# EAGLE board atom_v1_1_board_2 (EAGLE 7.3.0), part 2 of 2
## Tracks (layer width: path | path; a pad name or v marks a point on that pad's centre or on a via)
+3V3  (via drill 0.3)
  Top 0.152: 21.79,90.22 20.27,90.22 19.96,89.92 C9.+ 19.89,89.84 19.89,87.4 16.08,83.59 v16.08,83.21 | 21.79,90.22 25,90.22 C7.1 | 21.79,90.22 21.79,95.1 23.09,96.39 IC4.2 25.45,96.55 v26.29,97.38 | 12.35,75.89 13.34,75.89 15.32,77.88 17.76,77.88 18.52,78.64 SW3.B 18.59,78.72 v20.8,78.72 25.3,78.72 SW3.B' | 12.35,75.89 5.49,75.89 4.72,76.66 4.42,76.66 R45.2 | 68.89,78.03 68.89,79.25 R53.2 | 68.89,78.03 68.89,77.27 R52.2 68.81,77.19 68.5,77.19 v66.91,75.59 | 68.89,78.03 71.17,78.03 71.32,77.88 71.32,76.58 70.64,75.89 70.64,75.21 C39.1 70.56,75.13 v70.56,74.07 | 65.42,74.11 66.52,73 67.36,73 IC12.27 | 65.42,74.11 65.15,74.37 59.21,74.37 58.37,75.21 57.99,75.21 C38.1 | v58.29,73.08 58.83,73.61 59.82,73.61 IC12.1 | v57.46,74.07 57.46,74.75 57.84,75.13 C38.1 | v65.46,74.14 65.42,74.11 | 43.51,76.2 43.51,74.98 43.59,74.91 IC10.64 | 43.51,76.2 43.51,77.19 C21.1 43.51,77.27 v43.51,78.41 | C34.1 43.44,65.08 41.68,65.08 41.53,65.23 IC10.48 41.45,65.3 41.45,65.84 v40.84,66.45 | 12.35,75.89 12.35,73.99 12.5,73.84 21.95,73.84 23.7,75.59 27.05,75.59 29.11,73.53 29.11,73.46 C22.1 29.11,73.38 30.71,73.38 31.17,73.84 31.78,73.84 IC10.19 31.85,73.84 32.46,73.84 v33,73.3 | v33.07,63.17 32.92,63.02 32.01,63.02 C33.1 | v33,67.36 31.85,67.36 IC10.32 | 57.91,76.2 57.91,75.21 C38.1 | 57.91,76.2 57.91,77.19 C36.1 | v57,76.2 57.91,76.2 | 43.51,76.2 v44.35,76.2
  Bottom 0.152: v16.08,83.21 16.08,80.16 17.53,78.72 v20.8,78.72 | v58.29,73.08 58.29,73.23 v57.46,74.07 | v65.46,74.14 v66.91,75.59 | v33.07,63.17 33.07,67.28 v33,67.36 32.31,68.05 32.31,70.56 32.77,71.02 33,71.02 | v40.84,66.45 39.32,66.45 34.75,71.02 33,71.02 | v33,73.3 33,71.02 | v57,76.2 50.45,76.2 50.06,75.82 44.73,75.82 v44.35,76.2 | v43.51,78.41 43.51,81.38 45.03,82.91 45.03,83.06 JP1.1 | v26.29,97.38 30.33,97.38 34.14,101.19 52.81,101.19 53.34,101.73 66.91,101.73 70.56,98.07 v70.56,74.07
+3V3_A  (via drill 0.3)
  Top 0.152: C23.1 10.9,69.04 10.9,65.61 10.36,65.08 8.15,65.08 7.85,64.77 7.85,62.71 10.9,59.66 10.9,57.45 C29.1 10.9,57.38 v10.9,56.16 | v7.16,52.43 8.23,51.36 8.69,51.36 IC6.4 | v11.81,64.85 13.87,66.9 14.4,66.9 IC9.8 14.48,66.98 20.96,73.46 v23.47,73.46 | 32.01,78.94 32.01,79.25 C18.1 32.01,78.94 | 32.01,78.94 32.01,77.27 C17.1 | 32.01,78.94 34.82,78.94 | 34.82,78.94 35.13,78.94 35.59,78.49 35.59,78.03 35.51,77.95 35.51,77.11 IC10.13 | IC2.2 52.81,96.47 50.29,93.95 50.29,93.34 50.9,92.73 50.9,90.3 C8.1 50.83,90.3 v49.91,89.38 49.91,88.54 49.23,87.86 49.23,86.03 53.72,81.53 v53.72,73.08 | v34.82,79.25 34.82,78.94 | v54.26,89.84 C10.+ | 60.69,57.11 58.98,55.4 58.98,49.91 59.44,49.45 61.65,49.45 61.8,49.61 61.8,50.52 61.04,51.28 60.58,51.28 IC13.4 | 60.69,57.11 61.42,57.84 61.88,57.84 62.26,57.45 62.71,57.45 C51.1 | C48.1 57.91,61.49 57.91,63.48 C46.1 57.99,63.48 58.14,63.48 59.4,64.73 | 59.4,64.73 59.82,65.15 IC12.14 | v58.29,68.35 58.98,69.04 59.82,69.04 IC12.8 | 59.4,64.73 v58.29,65.84 | v60.66,57.23 60.66,57.15 60.69,57.11 | v48.31,39.55 47.17,39.55 IC3.16 | v48.31,40.92 45.87,40.92 45.84,40.96 | 45.84,40.96 45.19,41.6 C13.1 | IC5.16 47.17,30.33 49.15,30.33 49.61,30.79 49.61,31.24 48.39,32.46 45.19,32.46 C37.1 | 45.84,40.96 45.8,40.92 45.8,36.04 45.19,35.43 45.19,32.54 C37.1 | v53.27,36.27 57,32.54 57.23,32.54 JP102.1 | v36.88,56.01 36.88,57.38 C32.1 | v36.88,54.1 36.88,53.11 35.13,51.36 34.67,51.36 IC7.4 35.43,51.59 v36.27,50.75 | 32.5,41.11 32.01,41.6 C6.1 | 32.5,41.11 33.91,39.7 33.91,39.55 IC8.16 33.99,39.47 34.37,39.47 35.81,38.02 35.81,32.46 | C16.1 32.01,32.46 33.91,30.56 33.91,30.4 IC11.16 33.99,30.33 34.44,30.33 34.48,30.29
  Top 0.152: 34.48,30.29 36.42,28.35 36.42,26.29 28.73,18.59 17.76,18.59 14.78,15.62 13.87,15.62 R60.2 | 35.81,32.46 35.81,31.62 34.48,30.29 | 32.5,41.11 v33.07,41.68 | 35.81,32.46 40.92,32.46 42.75,30.63 43.74,30.63 45.19,32.08 45.19,32.38 C37.1
  Bottom 0.152: v7.16,52.43 v10.9,56.16 11.81,57.07 v11.81,64.85 | v54.26,89.84 50.37,89.84 v49.91,89.38 45.26,89.38 35.13,79.25 v34.82,79.25 34.44,78.87 28.88,78.87 v23.47,73.46 | v48.31,39.55 v48.31,40.92 52.81,40.92 53.23,40.5 | v53.27,36.27 53.27,40.46 53.23,40.5 | 53.23,40.5 53.27,40.54 53.8,40.54 60.66,47.4 v60.66,57.23 60.66,57.68 58.29,60.05 v58.29,65.84 v58.29,68.35 58.29,68.5 v53.72,73.08 | v36.88,54.1 v36.88,56.01 | v36.27,50.75 36.27,46.25 33.07,43.05 v33.07,41.68
ADC_ADDR_0  (via drill 0.3)
  Top 0.152: v32.84,27.13 33.91,27.13 IC11.11 | v32.84,35.59 33.53,36.27 33.91,36.27 IC8.11 | v45.34,27.13 47.09,27.13 IC5.11 | v48.24,35.97 47.93,36.27 47.17,36.27 IC3.11 | v36.5,75.59 36.88,75.21 38.71,75.21 39.93,76.43 39.93,77.04 IC10.4 | v29.41,64.01 29.41,62.41 33.53,58.29 34.9,58.29 36.12,57.07 36.12,55.85 38.1,53.87 v38.1,50.75
  Bottom 0.152: v32.84,35.59 32.84,32.31 | 32.84,32.31 v32.84,27.13 | 32.84,32.31 34.67,32.31 38.63,28.35 40.08,28.35 40.69,28.96 40.69,29.41 43.28,32 43.74,32 44.2,31.55 44.2,31.09 42.98,29.87 42.98,26.9 43.44,26.44 43.89,26.44 44.58,27.13 v45.34,27.13 46.71,28.5 46.71,34.44 v48.24,35.97 48.16,35.97 47.02,37.11 47.02,41.83 v38.1,50.75 | v36.5,75.59 34.06,75.59 33.53,75.06 33.38,75.06 31.01,72.69 31.01,65.61 v29.41,64.01
ADC_ADDR_1  (via drill 0.3)
  Top 0.152: v35.05,26.82 34.75,26.52 33.99,26.52 IC11.10 | v34.44,31.62 34.44,34.44 34.67,34.67 34.67,35.28 34.37,35.59 33.99,35.59 IC8.10 | v46.03,26.44 47.09,26.44 IC5.10 | v48.24,34.98 47.63,35.59 47.17,35.59 IC3.10 | v40.54,70.94 40.54,77.04 IC10.3 | v50.06,64.47 50.75,63.78 50.75,56.77 v47.93,53.95 | v40.39,26.82 v38.48,26.82
  Bottom 0.152: v34.44,31.62 34.44,27.58 35.05,26.98 v35.05,26.82 v38.48,26.82 | v40.54,70.94 40.54,70.18 45.03,65.68 48.84,65.68 v50.06,64.47 | v47.93,53.95 47.93,44.73 47.32,44.12 47.32,37.8 48.92,36.2 48.92,35.66 v48.24,34.98 47.55,34.29 47.55,28.88 46.03,27.36 v46.03,26.44 45.72,26.14 43.28,26.14 42.6,26.82 v40.39,26.82
ADC_ADDR_2  (via drill 0.3)
  Top 0.152: v32.84,26.14 33.07,25.91 33.91,25.91 IC11.9 | v32.16,33.68 32.62,33.68 33.91,34.98 IC8.9 | v48.24,26.21 47.93,25.91 47.17,25.91 IC5.9 | v48.24,33.91 47.17,34.98 IC3.9 | v44.35,84.89 41,81.53 41,77.11 IC10.2 | v54.41,71.48 v54.41,81.61 | v52.58,40.23 v53.57,41.22 | v40.08,24 45.19,24 v45.42,23.77
  Bottom 0.152: v32.16,33.68 32.16,26.82 v32.84,26.14 37.95,26.14 v40.08,24 | 48.24,33.83 v48.24,26.21 45.8,23.77 v45.42,23.77 | v44.35,84.89 51.13,84.89 v54.41,81.61 | v54.41,71.48 54.41,69.95 57.61,66.75 57.61,52.96 59.67,50.9 59.67,47.17 53.72,41.22 v53.57,41.22 | v52.58,40.23 52.58,38.18 48.24,33.83 | 48.24,33.83 v48.24,33.91
ADC_BANK_0  (via drill 0.3)
  Top 0.152: v27.2,27.05 27.28,27.13 28.27,27.13 IC11.6 | v42.52,51.44 43.97,51.44 44.43,51.89 44.43,52.96 44.73,53.26 49.38,53.26 52.27,56.16 52.58,56.16 54.79,58.37 54.79,65.91 v58.29,69.42 | v48.16,73.99 45.57,71.4 43.66,71.4 IC10.57
  Bottom 0.152: v27.2,27.05 27.2,28.88 25.83,30.25 25.83,38.48 27.28,39.93 31.39,39.93 32.39,40.92 32.39,47.78 36.04,51.44 v42.52,51.44 | v58.29,69.42 53.72,73.99 v48.16,73.99
ADC_BANK_1  (via drill 0.3)
  Top 0.152: v26.52,38.25 26.52,37.34 27.51,36.35 28.27,36.35 IC8.6 | v38.02,45.11 45.95,45.11 47.93,47.09 47.93,50.9 v49.3,52.27 | v55.48,58.45 v51.05,54.03 | v46.56,73.3 45.19,71.93 43.66,71.93 IC10.58
  Bottom 0.152: v26.52,38.25 31.17,38.25 v38.02,45.11 | v51.05,54.03 v49.3,52.27 | v55.48,58.45 55.48,68.43 50.6,73.3 v46.56,73.3
ADC_BANK_2  (via drill 0.3)
  Top 0.152: v39.7,29.34 39.7,28.57 41.07,27.2 41.45,27.2 IC5.6 | v43.28,42.82 47.4,42.82 v51.36,46.79 | v52.35,65 v52.35,56.84 | v44.96,72.62 44.5,72.62 44.27,72.39 43.66,72.39 IC10.59
  Bottom 0.152: v39.7,29.34 39.7,34.37 42.6,37.26 42.6,42.14 v43.28,42.82 | v51.36,46.79 51.36,47.24 52.35,48.23 v52.35,56.84 | v52.35,65 52.35,65.15 52.96,65.76 52.96,69.88 50.22,72.62 v44.96,72.62
ADC_BANK_3  (via drill 0.3)
  Top 0.152: v40.31,36.35 41.45,36.35 IC3.6 | v36.65,42.75 35.74,42.75 33.68,44.81 30.25,44.81 29.41,45.64 29.41,47.24 28.8,47.85 v28.8,48.84 | v41.07,57.23 45.57,57.23 49.07,60.73 49.07,66.98 v49.45,67.36 | v42.44,72.77 42.98,73.3 43.59,73.3 IC10.61
  Bottom 0.152: v40.31,36.35 40.31,39.09 v36.65,42.75 | v28.8,48.84 37.19,57.23 v41.07,57.23 | v49.45,67.36 47.85,67.36 v42.44,72.77
ADC_BLOW_SHAPE  (via drill 0.3)
  Top 0.152: R12.1 19.28,46.25 19.28,48.23 C15.2 | v33.07,77.34 33.3,77.11 33.91,77.11 IC10.16 | v24.46,73.53 24.46,72.62 25.83,71.25 25.83,70.79 22.86,67.82 v22.86,66.22 | v20.5,49.53 19.28,48.31 C15.2 | IC6.8 14.94,47.55 15.47,47.55 16.99,49.07 18.44,49.07 19.2,48.31 C15.2
  Bottom 0.152: v33.07,77.34 28.27,77.34 v24.46,73.53 | v22.86,66.22 22.86,51.89 v20.5,49.53
ADC_BLOW_TIMBRE  (via drill 0.3)
  Top 0.152: 6.1,47.47 6.1,48.23 C27.2 | 6.1,47.47 6.1,47.24 | 6.1,47.24 6.1,46.25 R35.1 | v39.85,74.91 31.85,74.91 IC10.17 | v16.77,80.39 12.96,80.39 v11.96,79.4 | 6.1,47.24 v5.18,47.24 | 6.1,47.47 8.69,47.47 IC6.7
  Bottom 0.152: v39.85,74.91 42.75,74.91 43.36,75.51 57.23,75.51 59.67,77.95 59.67,87.02 56.16,90.53 40.92,90.53 30.79,80.39 v16.77,80.39 | v11.96,79.4 11.96,65.91 5.18,59.13 v5.18,47.24
ADC_BOW_TIMBRE  (via drill 0.3)
  Top 0.152: R11.1 19.28,55.17 | 19.28,55.17 19.28,54.41 C14.2 | v33,76.35 33.15,76.2 34.22,76.2 34.44,76.43 34.44,77.04 IC10.15 | v25.15,71.02 25.15,70.79 v21.26,66.9 | v19.51,57.53 19.51,56.62 R11.1 | R11.1 | 19.28,55.17 14.94,55.17 IC6.14
  Bottom 0.152: v33,76.35 31.85,76.35 28.73,73.23 27.36,73.23 v25.15,71.02 | v21.26,66.9 20.35,66.9 19.51,66.06 v19.51,57.53
ADC_BRIGHTNESS  (via drill 0.3)
  Top 0.152: C42.2 71.1,48.23 71.1,46.25 R49.1 71.02,46.18 71.02,45.64 69.8,44.42 69.34,44.42 67.51,46.25 67.51,46.71 66.75,47.47 IC13.8 66.68,47.55 66.37,47.85 v65.08,47.85 | v33,70.33 31.85,70.33 IC10.26 | v58.98,47.4 59.67,46.71 v64.39,46.71
  Bottom 0.152: v33,70.33 33.15,70.33 39.02,64.47 44.73,64.47 51.66,57.53 52.58,57.53 58.98,51.13 v58.98,47.4 | v64.39,46.71 64.39,47.17 v65.08,47.85
ADC_DAMPING  (via drill 0.3)
  Top 0.152: R18.1 43.51,46.25 43.51,48.23 C20.2 43.44,48.23 v42.52,49.15 42.67,48.92 41.3,47.55 40.84,47.55 IC7.8 | v37.95,72.31 31.85,72.31 IC10.22 | v50.06,63.48 50.06,57.07 v46.94,53.95
  Bottom 0.152: v37.95,72.31 44.88,65.38 48.16,65.38 v50.06,63.48 | v46.94,53.95 46.94,53.57 v42.52,49.15
ADC_FM  (via drill 0.3)
  Top 0.152: 19.43,68.43 17.45,68.43 C25.2 17.38,68.35 17.38,68.12 14.94,65.68 14.48,65.68 IC9.7 | v30.25,75.67 35.66,75.67 36.42,76.43 36.42,77.04 IC10.11 | v24,72.16 23.17,72.16 19.43,68.43 | 19.43,68.43 R28.1
  Bottom 0.152: v30.25,75.67 27.51,75.67 v24,72.16
ADC_GEOMETRY  (via drill 0.3)
  Top 0.152: 32.01,47.47 32.01,48.23 C28.2 31.93,48.31 v32.84,49.23 | 32.01,47.47 32.01,46.25 R29.1 | v35.36,69.49 33,71.86 31.85,71.86 IC10.23 | v46.1,64.01 46.1,62.48 44.2,60.58 v42.29,60.58 | 32.01,47.47 34.6,47.47 IC7.7
  Bottom 0.152: v35.36,69.49 35.36,68.58 39.17,64.77 45.34,64.77 v46.1,64.01 | v42.29,60.58 42.29,55.17 38.86,51.74 35.36,51.74 v32.84,49.23
ADC_POSITION  (via drill 0.3)
  Top 0.152: C41.2 71.1,54.41 71.1,56.39 R48.1 71.02,56.39 71.02,57.23 66.68,61.57 64.16,61.57 63.32,60.73 63.32,60.43 63.25,60.35 v59.67,60.35 | v39.85,72.62 36.04,68.81 35.13,68.81 34.67,69.27 34.67,69.57 33.22,71.02 32.77,71.02 32.69,70.94 31.85,70.94 IC10.25 | v61.65,57.15 63.63,55.17 66.68,55.17 IC13.14
  Bottom 0.152: v39.85,72.62 41.38,72.62 43.44,74.68 53.95,74.68 59.67,68.96 v59.67,60.35 59.67,59.13 v61.65,57.15
ADC_POTS  (via drill 0.3)
  Top 0.152: v38.18,80.92 37.72,81.38 TP1.P$1 37.72,87.55 41.84,91.67 43.59,91.67 43.89,91.97 43.89,93.12 44.05,93.27 45.26,93.27 48.92,89.61 48.92,85.88 50.98,83.82 v50.98,70.41 | v36.81,80.01 37.26,80.01 37.95,79.32 37.95,77.11 IC10.8 | v27.13,29.87 27.89,29.11 28.27,29.11 IC11.3 | v27.2,37.57 27.81,38.18 28.27,38.18 IC8.3 | v38.25,31.77 41.15,31.77 42.29,30.63 42.29,29.49 41.91,29.11 41.53,29.11 IC5.3 | v43.28,37.19 42.33,38.14 | 42.33,38.14 42.29,38.18 41.53,38.18 IC3.3 | v51.66,67.67 49.38,65.38 49.38,57.3 v48.62,56.54 | v48.62,47.32 44.81,43.51 43.05,43.51 42.37,42.82 42.37,38.18 42.33,38.14
  Bottom 0.152: v38.18,80.92 37.72,80.92 v36.81,80.01 | v27.13,29.87 27.13,34.75 26.44,35.43 26.44,36.8 v27.2,37.57 27.2,37.49 27.43,37.26 32.77,37.26 v38.25,31.77 38.25,29.87 39.47,28.65 39.93,28.65 40.39,29.11 40.39,29.57 43.28,32.46 v43.28,37.19 | v50.98,70.41 50.98,68.66 51.66,67.97 v51.66,67.67 | v48.62,47.32 v48.62,56.54
ADC_PRESSURE  (via drill 0.3)
  Top 0.152: C26.2 4.34,54.41 4.34,56.39 R34.1 4.65,56.39 5.49,57.23 6.63,57.23 IC6.1 9.14,54.71 v10.36,54.71 | v34.9,78.26 34.9,77.11 IC10.14 | v28.8,72.24 28.2,72.24 v23.55,67.59
  Bottom 0.152: v34.9,78.26 34.9,77.34 33.22,75.67 32.23,75.67 v28.8,72.24 | v23.55,67.59 20.57,67.59 12.12,59.13 12.12,56.46 v10.36,54.71
ADC_SPACE  (via drill 0.3)
  Top 0.152: R73.1 56.16,46.25 56.16,48.23 C50.2 | v33.07,69.19 32.46,69.8 31.85,69.8 IC10.27 | v51.36,48.62 55.7,48.62 56.08,48.23 C50.2 | IC13.7 60.5,47.55 59.97,47.55 58.45,49.07 57,49.07 56.24,48.31 C50.2
  Bottom 0.152: v33.07,69.19 33.07,68.2 36.42,64.85 36.42,63.78 36.88,63.32 37.64,63.32 38.18,63.86 39.93,63.86 46.56,57.23 48.84,57.23 51.74,54.33 51.74,49 v51.36,48.62
ADC_STRIKE_SHAPE  (via drill 0.3)
  Top 0.152: 30.25,56.39 30.25,55.17 | 30.25,55.17 30.25,54.41 C30.2 | v27.13,66.22 28.2,67.28 28.2,70.33 31.17,73.3 31.78,73.3 IC10.20 | 30.25,56.39 v27.13,59.51 | 30.25,56.39 R46.1 | 30.25,55.17 34.6,55.17 IC7.1
  Bottom 0.152: v27.13,59.51 v27.13,66.22
ADC_STRIKE_TIMBRE
  Top 0.152: C19.2 43.51,54.41 43.51,56.39 R17.1 40.77,56.39 | 40.77,56.39 40.77,55.17 IC7.14 | 40.77,56.39 40.77,56.62 33.53,63.86 31.7,63.86 31.17,64.39 31.17,66.22 29.57,67.82 29.57,71.25 31.17,72.85 31.78,72.85 IC10.21
ADC_V_OCT  (via drill 0.3)
  Top 0.152: 4.19,68.43 6.17,68.43 C24.2 6.25,68.35 7.62,66.98 9.14,66.98 IC9.1 | v32.46,82.98 36.96,78.49 36.96,77.11 IC10.10 | v10.21,84.51 3.28,77.57 3.28,69.34 4.19,68.43 | 4.19,68.43 R27.1
  Bottom 0.152: v32.46,82.98 17.22,82.98 15.7,84.51 v10.21,84.51
AREF_-10
  Top 0.152: R32.2 4.34,50.29 4.34,52.27 R31.2 4.34,52.35 3.58,53.11 3.58,57 6.13,59.55 | 6.13,59.55 6.17,59.59 6.17,62.64 R37.2 | 30.25,50.29 30.25,52.27 R41.2 | 19.28,51.51 19.28,52.27 R14.2 19.28,52.35 20.19,53.26 20.19,57.76 17.45,60.5 17.45,62.64 R38.2 | 19.28,51.51 R15.2 | R15.2 29.49,50.29 | 29.49,50.29 30.25,50.29 | 30.25,50.29 R42.2 | R15.2 | 19.28,51.51 16.99,51.51 16.61,51.89 13.87,51.89 13.64,52.12 13.64,52.35 6.48,59.51 6.17,59.51 6.13,59.55 | C2.1 70.64,92.96 70.64,88.32 IC1.2 70.64,88.24 70.64,85.88 R2.2 70.56,85.8 R1.2 70.64,83.82 70.64,80.62 74.3,76.96 74.3,56.16 71.25,53.11 71.02,53.11 70.98,53.07 | R56.2 71.1,50.29 71.1,52.27 R55.2 71.02,52.35 71.02,53.03 70.98,53.07 | 45.19,50.29 45.19,52.27 R20.2 45.26,52.27 45.95,52.96 49.53,52.96 52.2,50.29 R70.2 56.24,50.29 56.24,53.72 60.73,58.22 63.4,58.22 63.55,58.06 63.55,56.92 63.86,56.62 65.08,56.62 65.69,57.23 69.95,57.23 70.18,57 70.18,53.87 70.98,53.07 | 29.49,50.29 29.49,47.62 30.1,47.02 30.86,47.02 31.17,46.71 31.17,45.64 31.39,45.41 35.43,45.41 35.81,45.8 42.52,45.8 42.9,45.41 45.8,45.41 45.95,45.57 45.95,49.53 45.19,50.29 | 45.19,50.29 R21.2
BOOT_FLASH  (via drill 0.3)
  Top 0.152: R50.2 17.3,76.66 17.3,75.97 18.52,74.75 SW3.A 18.59,74.68 20.65,74.68 v20.8,74.52 | v48.16,77.8 48.16,76.73 44.35,72.92 43.66,72.92 IC10.60 | v27.59,72.54 25.38,74.75 SW3.A'
  Bottom 0.152: v48.16,77.8 48.16,78.26 51.28,81.38 51.28,83.13 50.52,83.9 43.05,83.9 35.05,75.89 33.91,75.89 33.38,75.36 32.84,75.36 29.03,71.55 28.58,71.55 v27.59,72.54 27.59,72.47 25.45,70.33 24.92,70.33 23.32,71.93 23.32,72.01 v20.8,74.52
GATE  (via drill 0.3)
  Top 0.152: Q2.3 13.87,11.28 13.87,13.87 R60.1 13.95,13.87 v16,15.93 | v30.25,70.41 31.17,71.32 31.78,71.32 IC10.24 | v26.06,66.22 v27.51,67.67 | v20.5,44.81 20.5,44.65 16,40.16 v16,34.52
  Bottom 0.152: v27.51,67.67 v30.25,70.41 | v26.06,66.22 26.06,50.37 v20.5,44.81 | v16,15.93 v16,34.52
GND  (via drill 0.3)
  Top 0.152: IC12.15 67.44,65.15 69.04,63.55 69.34,63.55 C47.2 69.42,63.48 69.72,63.48 70.49,62.71 72.09,62.71 72.92,63.55 72.92,65.23 68.31,69.84 | 67.78,74.11 67.36,73.69 IC12.28 67.29,73.69 66.83,73.69 61.49,79.02 56.16,79.02 | 67.78,74.11 68.81,75.13 C39.2 | 68.31,69.84 69.65,71.17 69.65,72.24 67.78,74.11 | 68.31,69.84 68.28,69.8 67.44,69.8 IC12.22 67.36,69.72 67.36,69.11 IC12.21 67.29,69.11 62.71,69.11 60.81,67.21 59.89,67.21 IC12.11 59.82,67.13 58.67,67.13 56.24,64.69 56.24,63.55 C46.2 56.16,63.48 56.16,61.49 C48.2 56.24,61.42 57.99,59.66 64.54,59.66 | 64.54,59.66 64.54,60.12 65.38,60.96 C52.- | 64.54,59.66 64.54,57.45 C51.2 | C35.2 45.19,63.02 45.19,65 C34.2 45.19,65.08 45.19,66.22 48.69,69.72 51.89,69.72 52.96,70.79 54.64,70.79 56.16,72.31 56.16,75.13 C38.2 56.16,75.21 56.16,77.19 C36.2 56.16,77.27 56.16,79.02 | IC10.63 44.27,74.37 45.11,75.21 45.11,77.19 C21.2 45.19,77.27 45.19,78.49 46.03,79.32 46.03,79.78 44.27,81.53 44.27,83.44 44.73,83.9 45.57,83.9 46.33,83.13 JP1.3 46.41,83.13 47.63,83.13 | 68.81,89.92 68.81,88.32 IC1.1 | 68.81,89.92 68.81,92.96 C2.2 | 63.63,89.92 68.81,89.92 | 52.47,88.51 56.01,84.96 C10.- 56.01,84.89 56.16,84.73 56.16,79.02 | 52.47,88.51 52.43,88.54 50.98,88.54 C8.2 50.98,88.47 50.14,87.63 v50.14,87.48 | 54.26,91.82 54.26,90.75 52.5,89 52.5,88.54 52.47,88.51 | 54.26,91.82 54.26,97.23 52.88,98.6 52.88,98.75 IC2.1 52.81,98.83 49.07,98.83 48.46,99.44 42.06,99.44 40.39,97.77 P1.4 | 63.63,89.92 58.52,89.92 56.62,91.82 54.26,91.82 | 63.63,89.92 C1.+ | C31.2 30.25,65 30.25,63.02 C33.2 30.33,62.94 30.63,62.94 34.98,58.6 37.26,58.6 38.48,57.38 C32.2 38.56,57.38 38.56,53.72 38.48,53.65 38.48,53.19 39.09,52.58 IC7.12 40.84,52.58 40.84,51.36 IC7.11 40.84,51.28 40.84,50.06 IC7.10 40.77,50.06 34.67,50.06 IC7.5 34.6,50.06 34.22,50.06 33.38,50.9 33.38,51.74 34.22,52.58 IC7.3
  Top 0.152: v30.33,68.5 31.17,69.34 31.78,69.34 IC10.28 | 30.33,65.53 30.33,65.08 C31.2 | 30.33,65.53 v30.33,66.14 | 13.37,53.68 14.48,52.58 IC6.12 | 13.37,53.68 12.73,54.33 12.73,57.38 C29.2 12.65,57.45 12.65,63.17 | 10.71,64.96 10.14,64.39 IC9.3 | 10.71,64.96 12.65,66.9 12.65,69.04 C23.2 12.65,69.11 7.47,74.3 7.47,74.68 SW2.A 7.39,74.75 4.88,74.75 3.58,76.05 3.58,77.42 9.98,83.82 10.44,83.82 11.96,85.34 C3.- | IC9.3 9.22,63.17 IC9.4 | IC9.3 | 12.65,63.17 12.5,63.17 10.71,64.96 | 12.65,63.17 14.4,63.17 IC9.5 14.48,63.17 14.94,63.17 15.77,64.01 15.77,64.16 17.15,65.53 30.33,65.53 | 30.33,65.53 C31.2 | SW2.A' 14.25,74.75 15.47,75.97 15.47,76.66 R50.1 15.55,76.73 15.85,76.73 16.61,77.5 27.74,77.5 29.15,76.09 | 29.15,76.09 30.25,77.19 C17.2 30.25,77.27 30.25,79.25 C18.2 30.33,79.25 31.13,80.05 | 29.15,76.09 29.11,76.05 29.11,75.06 C22.2 29.19,75.06 29.87,74.37 31.78,74.37 IC10.18 | 31.13,80.05 31.17,80.09 34.9,80.09 35.97,79.02 35.97,77.11 IC10.12 | C3.- 12.35,84.96 15.24,82.07 C4.2 15.32,81.99 16.23,81.08 17.68,81.08 19.89,83.29 19.89,84.89 C9.- 19.96,84.96 23.55,88.54 25,88.54 C7.2 | C3.- 12.35,85.04 11.43,85.95 11.43,89.53 5.41,95.56 JP2.1 | 40.31,95.25 42.9,92.66 42.9,92.51 C12.1 | 40.31,95.25 40.31,97.77 P1.4 | 40.31,95.25 P1.3 | 37.72,97.77 35.2,97.77 | P1.5 36.92,94.45 | 36.92,94.45 36.88,94.41 36.88,92.51 C5.2 | 35.2,95.25 35.97,94.49 36.88,94.49 36.92,94.45 | 35.2,95.25 35.2,97.77 | 35.2,97.77 P1.8 | 35.2,95.25 P1.7 35.13,95.25 32.54,92.66 32.54,92.51 C11.1 32.54,92.73 31.93,92.73 31.39,93.27 28.2,93.27 25.8,90.87 | 37.72,97.77 40.23,97.77 P1.4 | 37.72,97.77 P1.6 | IC4.1 23.09,93.57 25.8,90.87
  Top 0.152: 25.8,90.87 25.83,90.83 25.83,89.38 25.07,88.62 C7.2 | 31.13,80.05 31.09,80.09 31.09,82.37 25,88.47 C7.2 | 47.55,5.87 47.55,7.09 C54.2 | 47.55,5.87 47.55,5.11 R74.1 | 47.55,5.87 44.58,5.87 44.27,5.56 44.27,3.81 43.51,3.05 R59.1 42.52,3.05 40.39,5.18 IC14.5 40.31,5.18 38.63,3.5 38.63,3.05 C45.1 38.56,3.05 37.57,2.06 36.2,2.06 33.26,4.99 | 33.26,4.99 33.6,5.33 33.6,5.64 34.44,6.48 IC14.3 | 33.26,4.99 32.04,3.77 | 32.04,3.77 32.01,3.73 32.01,3.05 R69.1 | 27.89,5.87 27.89,7.09 C57.2 27.97,7.16 27.97,8.23 28,8.27 | 27.89,5.87 27.89,5.11 R87.1 | 28,8.27 30.86,11.12 36.81,11.12 C44.2 36.88,11.2 v36.88,14.48 | Q2.2 14.86,8.99 17.15,8.99 17.83,8.31 27.97,8.31 28,8.27 | 27.89,5.87 30.86,5.87 31.01,5.71 31.01,4.65 31.85,3.81 32.01,3.81 32.04,3.77 | IC6.10 14.94,50.06 14.94,51.28 IC6.11 14.86,51.28 v13.26,51.28 9.98,51.28 | 9.98,51.28 9.98,51.74 9.14,52.58 IC6.3 | 9.98,51.28 9.98,50.83 9.22,50.06 8.76,50.06 IC6.5 9.3,50.06 9.98,49.38 9.98,47.02 5.26,42.29 5.26,40.16 JP3.1 | IC5.7 41.53,26.44 41.53,25.91 IC5.8 41.45,25.83 v40.39,25.83 | IC11.8 28.27,25.91 28.27,26.44 IC11.7 28.35,26.52 28.73,26.52 30.02,27.81 31.47,27.81 | 31.47,27.81 33.91,27.81 IC11.12 33.99,27.81 v35.13,27.81 | 31.47,27.81 31.47,28.8 30.33,29.95 30.33,32.46 C16.2 | IC8.8 28.27,35.05 28.27,35.59 IC8.7 28.35,35.66 28.73,35.66 29.03,35.97 29.03,36.58 28.73,36.88 28.35,36.88 IC8.5 28.27,36.96 28.27,37.57 IC8.4 28.35,37.64 28.73,37.64 29.03,37.95 29.03,38.56 28.73,38.86 28.35,38.86 IC8.2 | IC8.2 28.27,38.94 28.27,39.47 IC8.1 28.35,39.55 30.25,41.45 30.25,41.6 C6.2 30.33,41.68 30.56,41.68 31.32,42.44 33.3,42.44 40.08,35.66 41.45,35.66 IC3.7
  Top 0.152: IC3.7 41.53,35.59 41.53,35.05 IC3.8 41.53,34.98 43.44,33.07 43.44,32.54 C37.2 43.51,32.46 v43.51,31.32 | IC3.7 41.61,35.59 42.6,35.59 43.97,36.96 43.97,37.41 43.51,37.87 43.51,41.6 C13.2 43.59,41.6 43.74,41.6 44.58,42.44 54.94,42.44 57.23,40.16 JP6.1 57.3,40.08 65.23,40.08 | IC13.5 60.5,50.06 60.12,50.06 59.28,50.9 59.28,51.74 60.12,52.58 IC13.3 IC13.12 66.75,52.58 66.75,51.36 IC13.11 66.75,51.28 66.75,50.06 IC13.10 66.68,49.99 66.22,49.99 64.39,48.16 64.39,47.62 65.23,46.79 65.23,40.08 | 65.23,40.08 70.18,40.08 JP8.1 | JP4.1 18.14,40.08 18.14,39.24 16.99,38.1 16.99,37.03 17.6,36.42 23.77,36.42 26.29,38.94 28.2,38.94 IC8.2 | v13.26,53.65 13.34,53.65 13.37,53.68 | 47.63,83.13 48.35,83.86 | 48.35,83.86 48.39,83.9 49.23,83.9 49.99,83.13 50.14,83.13 JP1.9 | 47.63,83.13 JP1.5 | v48.31,85.65 48.31,83.9 48.35,83.86
  Bottom 0.152: v30.33,66.14 v30.33,68.5 | JP2.1 | JP4.1 18.14,40.16 5.26,40.16 JP3.1 | 39.21,27.01 38.41,27.81 v35.13,27.81 | 39.21,27.01 v40.39,25.83 40.77,25.45 40.77,17.91 37.34,14.48 v36.88,14.48 | v43.51,31.32 39.21,27.01 | JP103.1 57.3,37.64 57.3,40.08 JP6.1 | v13.26,51.28 v13.26,53.65 | v50.14,87.48 v48.31,85.65
  other vias: 13.97,18.8 25.15,20.07 28.19,23.11 41.66,20.83 44.7,17.02 61.47,34.54 63.25,28.7 61.47,14.73 48.01,14.22 54.36,15.49 47.24,9.4 13.46,36.83 22.61,38.61 27.43,41.66 51.82,43.43 54.36,52.58 55.63,56.39 26.16,47.24 4.57,60.71 24.64,61.21 24.64,52.58 64.52,78.23 62.23,96.52 26.16,81.79 66.55,82.55 53.85,18.54
  pour Bottom: 0,0 75.3,0 75.3,108 0,108
  pour Top: 0,0 75.3,0 75.3,108 0,108
I2C_SCL  (via drill 0.3)
  Top 0.152: v66.91,74.6 68.28,75.97 69.04,75.97 70.26,77.19 70.56,77.19 R52.1 | v65.84,71.48 66.07,71.48 66.45,71.09 67.36,71.09 IC12.24 | v41.76,73.91 41.76,71.25 40.77,70.26 37.95,70.26 36.2,68.5 32.84,68.5 32.54,68.81 31.85,68.81 IC10.29 | v62.18,75.21 v59.28,75.21
  Bottom 0.152: v66.91,74.6 66.91,72.54 v65.84,71.48 65.84,71.55 v62.18,75.21 | v41.76,73.91 42.22,73.91 43.51,75.21 v59.28,75.21
I2C_SDA  (via drill 0.3)
  Top 0.152: v71.63,74.07 71.63,78.03 70.64,79.02 70.64,79.25 R53.1 69.72,80.09 65.69,80.09 v57.46,88.32 | v68.96,71.4 68.96,71.09 68.28,70.41 67.44,70.41 IC12.23 | v32.39,66.6 33.15,66.6 33.68,67.13 33.68,67.59 33.22,68.05 32.84,68.05 32.54,68.35 31.85,68.35 IC10.30 | v48.24,87.86 v42.83,82.45
  Bottom 0.152: v68.96,71.4 v71.63,74.07 | v32.39,66.6 32.39,67.06 32.01,67.44 32.01,73.23 33.53,74.75 36.58,74.75 37.8,75.97 37.8,77.42 v42.83,82.45 | v48.24,87.86 49.23,87.86 49.68,88.32 v57.46,88.32
I2S_LRCK  (via drill 0.3)
  Top 0.152: v41.76,69.88 38.02,69.88 33.99,65.84 33.99,65.3 IC10.33 | v51.59,66.67 54.18,66.67 58.52,71.02 59.82,71.02 IC12.5 59.89,71.02 60.73,71.02 61.11,70.64 61.11,70.1 60.81,69.8 59.89,69.8 IC12.7
  Bottom 0.152: v41.76,69.88 44.88,69.88 48.08,66.67 v51.59,66.67
I2S_MCK
  Top 0.152: IC10.37 36.04,65.23 36.04,64.01 40.16,59.89 45.11,59.89 45.19,59.97 46.03,59.97 48.46,62.41 48.46,68.12 49.76,69.42 52.05,69.42 53.11,70.48 54.79,70.48 58.37,74.07 64.16,74.07 66.52,71.7 67.36,71.7 IC12.25
I2S_SCK  (via drill 0.3)
  Top 0.152: v46.41,58.98 46.03,58.6 40.46,58.6 34.52,64.54 34.52,65.23 IC10.34 | v45.8,60.66 45.8,61.72 46.79,62.71 v46.79,66.9 | v47.09,69.04 v45.95,67.89 | v50.67,68.05 51.13,68.05 53.27,70.18 56.77,70.18 58.9,72.31 59.82,72.31 IC12.3
  Bottom 0.152: v46.41,58.98 46.41,60.05 v45.8,60.66 | v46.79,66.9 46.79,67.06 v45.95,67.89 | v47.09,69.04 48.77,69.04 49.76,68.05 v50.67,68.05
I2S_SIN  (via drill 0.3)
  Top 0.152: v42.44,69.19 38.33,69.19 34.98,65.84 34.98,65.3 IC10.35 | v52.27,65.99 53.95,65.99 58.29,70.33 59.82,70.33 IC12.6
  Bottom 0.152: v42.44,69.19 43.59,69.19 46.79,65.99 v52.27,65.99
I2S_SOUT  (via drill 0.3)
  Top 0.152: v38.41,66.45 36.04,66.45 35.51,65.91 35.51,65.3 IC10.36 | v54.79,68.2 55.25,68.2 58.67,71.63 59.82,71.63 IC12.4
  Bottom 0.152: v38.41,66.45 38.86,66.45 40.23,65.08 47.55,65.08 49.84,62.79 51.05,62.79 54.79,66.52 v54.79,68.2
JTCK  (via drill 0.3)
  Top 0.152: v40.84,68.5 41.91,67.44 43.59,67.44 IC10.49
  Bottom 0.152: v40.84,68.5 37.26,72.08 37.26,73.23 41.76,77.72 43.74,77.72 44.65,78.64 44.65,80.16 46.33,81.84 JP1.4
JTDI
  Top 0.152: IC10.50 43.66,67.89 44.27,67.89 49.15,72.77 49.15,81.61 48.92,81.84 JP1.8
JTDO
  Top 0.152: IC10.55 43.66,70.41 45.49,70.41 48.84,73.76 48.84,80.62 47.63,81.84 JP1.6
JTMS  (via drill 0.3)
  Top 0.152: v42.14,62.56 40.54,64.16 40.54,65.23 IC10.46 | v45.42,59.28 45.8,59.28 48.77,62.26 48.77,67.59 49.91,68.73 v49.99,68.73 | v49.99,71.93 49.99,76.35 v49.84,76.5 | v46.33,78.72 46.33,80.62 45.11,81.84 JP1.2
  Bottom 0.152: v45.42,59.28 v42.14,62.56 | v49.99,71.93 v49.99,68.73 | v49.84,76.5 48.54,76.5 v46.33,78.72
LED_GATE  (via drill 0.3)
  Top 0.152: v49.76,36.27 52.05,33.98 52.05,30.02 R10.1 | v37.11,64.01 36.5,64.62 36.5,65.23 IC10.38
  Bottom 0.152: v49.76,36.27 49.76,37.19 47.63,39.32 47.63,43.97 52.05,48.39 52.05,55.32 43.21,64.16 37.26,64.16 v37.11,64.01
LIN  (via drill 0.3)
  Top 0.152: v72.16,64.77 68.5,68.43 67.44,68.43 IC12.20 | v20.73,4.04 19.74,3.05 C56.+
  Bottom 0.152: v72.16,64.77 72.92,64.01 72.92,10.67 70.56,8.31 68.35,8.31 64.08,4.04 v20.73,4.04
LOUT  (via drill 0.3)
  Top 0.152: v61.72,66.52 59.89,66.52 IC12.12 | v63.4,5.18 63.4,3.05 C40.+
  Bottom 0.152: v61.72,66.52 61.72,61.65 63.7,59.66 63.7,46.48 65.69,44.5 66.45,44.5 67.29,43.66 67.29,9.07 v63.4,5.18
N$1
  Top 0.305: D1.+ 28.12,98.15 32.31,98.15 32.62,97.84 P1.10 32.69,97.69 32.69,95.25 P1.9
N$2  (via drill 0.3)
  Top 0.152: R15.1 16.84,50.29 15.32,48.77 IC6.9 14.48,48.77 13.64,47.93 13.64,46.94 15.96,44.62 | v9.68,16.15 9.68,14.78 R16.1 | 15.96,44.62 17.53,46.18 R12.2 17.6,46.25 17.6,48.23 C15.1 | 15.96,44.62 v9.68,38.33
  Bottom 0.152: v9.68,38.33 v9.68,16.15
N$3
  Top 0.305: D2.- 47.85,94.87 43.21,94.87 42.83,95.25 P1.1 42.83,95.33 42.83,97.77 P1.2
N$4
  Top 0.152: R36.2 7.85,9.68 5.26,9.68 JP25.1
N$5  (via drill 0.3)
  Top 0.152: R11.2 14.48,56.39 13.64,55.55 13.64,54.63 14.4,53.87 14.86,53.87 IC6.13 14.94,53.87 17.07,53.87 17.53,54.33 C14.1 17.6,54.33 18.44,53.49 v18.44,53.34 17.6,52.5 17.6,52.35 R14.1 | v12.88,20.5 9.68,17.3 R13.1
  Bottom 0.152: v12.88,20.5 12.88,33.98 17.83,38.94 18.67,38.94 19.36,39.62 19.36,52.43 v18.44,53.34
N$6  (via drill 0.3)
  Top 0.305: v66.07,43.66 66.07,45.8 v66.68,46.41
  Bottom 0.305: JP107.1 57.46,35.05 v66.07,43.66 | v66.68,46.41 66.68,71.02 69.19,73.53 69.19,97.54 JP9.2
N$7
  Top 0.152: C12.2 44.65,92.43 44.65,90.45 42.6,88.39 Q1.2 42.52,88.39 39.47,85.34 39.47,77.11 IC10.5
N$8
  Top 0.152: C11.2 30.79,92.43 30.79,90.45 32.84,88.39 Q1.1 32.92,88.39 32.92,85.27 38.94,79.25 38.94,77.11 IC10.6
N$9  (via drill 0.3)
  Top 0.152: R17.2 45.19,56.39 45.19,54.41 C19.1 45.11,54.33 43.51,52.73 43.51,52.35 R20.1 43.51,52.81 42.29,52.81 41.3,53.8 40.84,53.8 IC7.13 40.77,53.8 40.39,53.42 v39.17,53.42 | v23.39,15.39 23.39,12.19 R19.1
  Bottom 0.152: v23.39,15.39 23.39,24.23 26.14,26.98 26.14,29.49 24.46,31.17 24.46,42.67 35.2,53.42 v39.17,53.42
N$10
  Top 0.152: JP26.1 R39.2
N$11
  Top 0.152: R27.2 4.19,66.75 6.17,66.75 C24.1 6.25,66.67 6.25,65.68 | R36.1 9.6,9.68 9.6,10.82 8.69,11.73 8.69,17.91 8,18.59 4.72,18.59 3.28,20.04 3.28,61.42 6.17,64.31 R37.1 6.25,64.39 6.25,65.68 | 6.25,65.68 9.14,65.68 IC9.2
N$13
  Top 0.152: C35.1 43.44,63.02 42.6,63.02 41,64.62 41,65.23 IC10.47
N$14  (via drill 0.3)
  Top 0.152: R18.2 45.19,46.25 45.19,48.23 C20.1 45.11,48.31 43.51,49.91 43.51,50.29 R21.1 43.51,49.84 42.29,49.84 41.23,48.77 IC7.9 40.39,48.77 39.55,47.93 39.55,47.02 v40.01,46.56 | v48.92,18.9 52.05,15.77 52.05,12.19 R22.1 | v53.57,27.58 53.11,27.58 49.91,30.79 49.91,31.39 48.08,33.22 47.85,33.22 v45.87,35.2
  Bottom 0.152: v48.92,18.9 48.92,22.94 v53.57,27.58 | v45.87,35.2 45.87,41.6 40.92,46.56 v40.01,46.56
N$15  (via drill 0.3)
  Top 0.152: IC9.6 14.94,64.39 17.22,66.67 17.38,66.67 C25.1 17.45,66.75 19.43,66.75 R28.2 19.43,66.67 20.12,66.67 v20.57,66.22 | R39.1 58.98,12.19 57.76,13.41 53.65,13.41 52.88,12.65 52.88,11.58 52.66,11.35 40.92,11.35 37.11,15.16 v24.39,15.16 | v20.5,52.65 20.5,61.27 17.45,64.31 R38.1
  Bottom 0.152: v24.39,15.16 24.08,15.16 23.62,14.71 23.17,14.71 19.81,18.06 19.81,51.97 v20.5,52.65 20.5,52.58 21.87,53.95 21.87,54.41 20.57,55.7 v20.57,66.22
N$17
  Top 0.152: C47.1 71.02,63.55 70.72,63.55 68.43,65.84 67.44,65.84 IC12.16 67.36,65.84 66.52,65.84 61.88,61.19 61.88,60.96 C52.+
N$18
  Top 0.152: R86.1 23.39,7.09 26.14,7.09 C57.1 26.14,7.01 26.14,5.11 R87.2 26.06,5.11 24,3.05 C56.-
N$19
  Top 0.152: C31.1 31.93,65.08 31.93,66.14 30.94,67.13 30.94,67.59 31.17,67.82 31.78,67.82 IC10.31
N$22
  Top 0.152: R75.1 52.05,7.09 49.3,7.09 C54.1 49.23,7.09 49.23,5.11 R74.2 49.3,5.03 51.28,3.05 C55.-
N$23
  Top 0.152: 45.19,3.05 45.19,5.03 R58.2 | 45.19,3.05 50.29,3.05 50.9,2.44 59.21,2.44 C40.- | 45.19,3.05 R59.2
N$24  (via drill 0.3)
  Top 0.152: R46.2 35.05,56.39 35.89,55.55 35.89,54.63 35.13,53.87 34.67,53.87 IC7.2 34.6,53.87 32.46,53.87 32.01,54.33 C30.1 31.93,54.33 31.2,53.61 | v22.02,10.97 23.32,9.68 R40.1 | v21.18,54.18 29.03,54.18 29.64,53.57 31.17,53.57 31.2,53.61 | 31.2,53.61 31.93,52.88 31.93,52.35 R41.1
  Bottom 0.152: v22.02,10.97 13.95,10.97 8.15,16.76 8.15,36.35 5.56,38.94 4.72,38.94 4.04,39.62 4.04,40.69 17.53,54.18 v21.18,54.18
N$25
  Top 0.152: 43.51,6.48 43.51,7.09 C43.1 43.51,7.16 43.51,9.14 R51.2 | 43.51,6.48 43.51,5.11 R58.1 | 43.51,6.48 IC14.6
N$27
  Top 0.152: R33.1 9.3,19.81 7.93,21.18 4.65,21.18 3.73,22.1 3.73,45.57 4.34,46.18 R35.2 4.34,46.25 4.34,48.23 C27.1 4.42,48.31 6.02,49.91 6.02,50.29 R32.1 6.02,49.84 7.09,48.77 IC6.6
N$28
  Top 0.152: 45.19,8.31 45.19,9.14 R51.1 45.11,9.14 44.27,9.98 42.9,9.98 42.67,9.75 42.67,9.37 41.07,7.77 40.39,7.77 IC14.7 | 45.19,8.31 45.19,7.16 C43.2 | 45.19,8.31 57.76,8.31 58.9,7.16 64.77,7.16 R88.2
N$30  (via drill 0.3)
  Top 0.152: v67.97,16.61 67.82,16.46 66.83,16.46 65.15,14.78 64.85,14.78 R57.1 | v69.57,45.11 69.57,46.02 69.42,46.18 R49.2 69.42,46.25 69.42,48.23 C42.1 | 69.42,48.77 69.42,48.31 C42.1 | 69.42,48.77 69.42,50.29 R56.1 | 69.42,48.77 IC13.9 | 69.42,48.77 C42.1
  Bottom 0.152: v67.97,16.61 67.97,26.9 69.88,28.8 70.79,28.8 72.09,30.1 72.09,42.6 v69.57,45.11
N$31
  Top 0.152: 30.25,3.05 30.25,5.03 R68.2 | 30.25,3.05 25.15,3.05 24.54,2.44 16.23,2.44 C53.- | 30.25,3.05 R69.2
N$32
  Top 0.152: R68.1 32.01,5.11 32.01,7.09 C49.1 32.01,7.16 32.01,7.77 | 32.01,7.77 32.01,9.14 R72.2 | 32.01,7.77 35.05,7.77 IC14.2
N$33
  Top 0.152: C49.2 30.25,7.16 30.25,9.14 R72.1 30.56,9.14 31.39,9.98 34.14,9.98 35.05,9.07 IC14.1 35.13,9.07 37.64,9.07 38.18,9.6 38.63,9.6 40.01,10.97 57.68,10.97 58.98,9.68 64.77,9.68 R89.2
N$35  (via drill 0.3)
  Top 0.152: IC13.6 59.67,48.77 58.14,50.29 R70.1 57.61,50.29 56.62,49.3 51.13,49.3 50.67,48.84 50.67,48.39 53.65,45.41 57.08,45.41 57.84,46.18 R73.2 | v63.7,17.91 64.31,17.3 64.77,17.3 R71.1 | v64.54,40.77 63.32,40.77 57.91,46.18 R73.2 | C50.1 57.91,48.23 57.91,46.25 R73.2
  Bottom 0.152: v63.7,17.91 63.7,18.97 66.98,22.25 66.98,38.33 v64.54,40.77
N$37  (via drill 0.3)
  Top 0.152: C28.1 30.33,48.31 30.33,48.69 31.93,50.29 R42.1 32.69,50.29 34.22,48.77 IC7.6 v39.17,48.77 | v50.98,10.29 51.59,9.68 52.05,9.68 R43.1 | v50.98,19.13 50.98,19.58 44.65,25.91 44.65,28.04 v46.03,29.41 | v36.04,45.11 31.24,45.11 30.33,46.02 30.33,46.18 R29.2
  Bottom 0.152: v50.98,19.13 v50.98,10.29 | v46.03,29.41 46.03,34.44 46.56,34.98 46.56,41.38 v39.17,48.77 39.4,48.46 v36.04,45.11
N$38
  Top 0.152: R10.2 53.87,29.95 57.23,29.95 JP95.1
N$40
  Top 0.152: R54.1 65.08,19.81 66.45,21.18 70.79,21.18 72.09,22.48 72.09,32.38 70.64,33.83 69.72,33.83 69.04,34.52 69.04,35.59 69.88,36.42 70.79,36.42 71.86,37.49 71.86,48.92 71.32,49.45 70.49,49.45 70.18,49.76 70.18,51.51 69.42,52.27 R55.1 69.42,52.35 69.42,53.87 | 69.42,53.87 69.42,54.33 C41.1 | R48.2 69.42,56.39 69.42,54.41 C41.1 | 69.42,53.87 66.75,53.87 IC13.13 | 69.42,53.87 C41.1
N$41
  Top 0.152: JP27.1 R30.2
N$42  (via drill 0.3)
  Top 0.152: 6.1,53.87 6.1,54.33 C26.1 | 6.1,53.87 6.1,52.35 R31.1 6.02,52.27 v6.93,51.36 | R34.2 6.1,56.39 6.1,54.41 C26.1 | v9.6,13.56 R30.1 | 6.1,53.87 8.69,53.87 IC6.2 | 6.1,53.87 C26.1
  Bottom 0.152: v9.6,13.56 9.6,14.55 5.56,18.59 4.72,18.59 3.73,19.58 3.73,44.88 6.93,48.08 v6.93,51.36
N$44
  Top 0.152: IC13.2 60.58,53.87 60.58,55.09 IC13.1
N$54  (via drill 0.3)
  Top 0.152: v20.5,31.85 20.65,31.7 22.25,31.7 23.01,32.46 23.32,32.46 R44.1 | v39.32,63.17 39.32,64.47 39.4,64.54 39.4,65.23 IC10.44
  Bottom 0.152: v20.5,31.85 20.5,43.89 33.99,57.38 33.99,57.84 v39.32,63.17
N$61  (via drill 0.3)
  Top 0.305: F1.1 23.32,102.11 23.32,99.06 IC4.3 23.39,98.98 v24.77,97.61 | v38.56,93.73 38.56,92.51 C5.1
  Bottom 0.305: v38.56,93.73 28.65,93.73 v24.77,97.61
N$66
  Top 0.152: R67.2 9.68,7.16 11.05,7.16 12.88,8.99 Q2.1
N$79  (via drill 0.3)
  Top 0.152: v25.15,36.8 23.39,35.05 R47.1 | v39.47,61.49 39.02,61.49 37.64,62.87 37.64,63.63 37.95,63.93 37.95,65.23 IC10.41
  Bottom 0.152: v25.15,36.8 25.15,42.9 34.98,52.73 39.4,52.73 41.76,55.09 41.76,59.21 v39.47,61.49
N$80  (via drill 0.3)
  Top 0.305: v18.67,83.82 18.67,83.74 16.99,82.07 C4.1 | v51.13,93.65 52.27,93.65 52.81,94.18 IC2.3 | v55.09,100.89 54.33,101.65 54.33,102.11 F2.1
  Bottom 0.305: v18.67,83.82 32.01,83.82 41.84,93.65 50.22,93.65 | v51.13,93.65 50.22,93.65 | v55.09,100.89 53.27,100.89 50.22,97.84 50.22,93.65
N$81
  Top 0.152: R75.2 53.87,7.09 57.23,7.09 JP5.1
N$82
  Top 0.152: R89.1 68.33,9.65 69.6,10.92 70.87,10.92 71.63,10.16 71.63,8.51 JP11.1
N$84
  Top 0.152: R88.1 66.8,7.11 69.34,9.65 JP10.1
N$86
  Top 0.152: R86.2 21.57,7.09 18.21,7.09 JP7.1
N$87
  Top 0.152: R13.2 7.85,17.3 5.26,17.3 JP28.1
N$88
  Top 0.152: R16.2 7.85,14.71 5.26,14.71 JP29.1
N$89
  Top 0.152: JP30.1 R33.2
N$93
  Top 0.152: R40.2 21.57,9.68 18.21,9.68 JP31.1
N$94
  Top 0.152: JP32.1 R19.2
N$95
  Top 0.152: JP33.1 R22.2
N$96
  Top 0.152: R43.2 53.87,9.68 57.23,9.68 JP34.1
N$97
  Top 0.152: R71.2 66.52,17.3 70.18,17.3 JP37.1
N$98
  Top 0.152: R57.2 66.52,14.71 70.18,14.71 JP36.1
N$99
  Top 0.152: JP35.1 R54.2
N$100  (via drill 0.3)
  Top 0.152: v30.71,21.95 31.09,21.95 35.81,26.67 35.81,28.04 35.36,28.5 33.99,28.5 IC11.13 | v66.3,33.76 70.18,37.64 JP65.1
  Bottom 0.152: v30.71,21.95 30.71,11.73 36.42,6.02 49.38,6.02 56.92,13.56 57.84,13.56 66.3,22.02 v66.3,33.76
N$101
  Top 0.152: JP66.1 6.4,23.7 23.77,23.7 26.21,21.26 30.94,21.26 36.12,26.44 36.12,28.19 35.28,29.03 33.99,29.03 IC11.14
N$102  (via drill 0.3)
  Top 0.152: v25.45,29.11 29.64,33.3 30.86,33.3 31.01,33.15 31.01,32.08 33.3,29.79 33.91,29.79 IC11.15 | v20.5,21.79 19.28,21.79 18.67,21.18 8.38,21.18 7.24,22.33 5.26,22.33 JP67.1
  Bottom 0.152: v25.45,29.11 25.45,26.75 v20.5,21.79
N$103  (via drill 0.3)
  Top 0.152: v30.79,28.57 29.03,30.33 28.35,30.33 IC11.1 | v40.08,23.01 46.18,23.01 v49.61,19.58
  Bottom 0.152: v30.79,28.57 30.79,26.44 34.22,23.01 v40.08,23.01 | v49.61,19.58 50.06,19.58 52.81,22.33 57.23,22.33 JP68.1
N$104
  Top 0.152: IC11.5 28.27,27.74 20.96,27.74 20.04,28.65 6.48,28.65 5.26,27.43 JP69.1
N$105  (via drill 0.3)
  Top 0.152: v29.41,29.03 28.73,29.72 28.35,29.72 IC11.2 | v24.08,22.48 18.29,22.48 JP70.1
  Bottom 0.152: v29.41,29.03 29.41,27.81 v24.08,22.48
N$106  (via drill 0.3)
  Top 0.152: v21.64,28.42 28.27,28.42 IC11.4 | v20.5,27.28 19.74,27.28 18.67,26.21 4.72,26.21 4.04,26.9 4.04,36.42 JP71.1
  Bottom 0.152: v20.5,27.28 v21.64,28.42
N$107
  Top 0.152: IC8.13 33.91,37.57 32.31,37.57 31.09,36.35 31.01,36.35 29.34,34.67 29.34,34.52 24.84,30.02 18.21,30.02 JP72.1
N$108  (via drill 0.3)
  Top 0.152: v31.17,40.62 33.53,38.25 33.91,38.25 IC8.14 | v27.74,44.58 21.18,44.58 17.91,41.3 17.6,41.3 16.69,40.39 v16.69,35.74
  Bottom 0.152: v31.17,40.62 31.17,41.15 v27.74,44.58 | v16.69,35.74 16.69,21.26 18.14,19.81 JP73.1
N$109  (via drill 0.3)
  Top 0.152: v35.13,33.98 35.13,38.1 34.37,38.86 33.99,38.86 IC8.15
  Bottom 0.152: v35.13,33.98 35.13,34.21 33.07,36.27 32.62,36.27 31.93,35.59 31.93,34.37 30.1,32.54 30.1,23.47 34.52,19.05 34.52,8.38 36.58,6.33 37.26,6.33 50.75,19.81 JP74.1
N$110  (via drill 0.3)
  Top 0.152: v31.24,35.66 32.46,36.88 33.91,36.88 IC8.12 | v27.13,35.66 25.38,35.66 23.55,33.83 v7.47,33.83
  Bottom 0.152: v27.13,35.66 v31.24,35.66 | v7.47,33.83 6.48,33.83 5.26,35.05 JP75.1
N$111
  Top 0.152: IC5.13 47.17,28.42 47.55,28.42 56.08,19.89 56.08,19.28 56.77,18.59 70.72,18.59 72.39,20.27 72.39,32.92 70.26,35.05 JP76.1
N$112
  Top 0.152: IC5.14 47.17,29.03 48.92,29.03 56.77,21.18 65.99,21.18 67.13,22.33 70.18,22.33 JP77.1
N$113
  Top 0.152: JP78.1 69.04,23.7 55.17,23.7 49.15,29.72 47.17,29.72 IC5.15
N$114  (via drill 0.3)
  Top 0.152: v46.1,25.38 48.31,25.38 48.92,25.98 48.92,26.44 47.63,27.74 47.17,27.74 IC5.12 | v43.05,22.33 34.29,22.33 28.04,16.08 21.64,16.08 v21.26,15.7
  Bottom 0.152: v43.05,22.33 v46.1,25.38 | v21.26,15.7 21.26,16.15 19.36,18.06 19.36,26.29 18.21,27.43 JP79.1
N$115
  Top 0.152: IC5.1 41.45,30.33 39.32,30.33 36.73,27.74 36.73,26.14 27.89,17.3 18.21,17.3 JP80.1
N$116
  Top 0.152: IC5.5 41.53,27.81 43.89,27.81 44.35,27.36 44.35,25.76 50.29,19.81 50.29,18.9 51.89,17.3 57.23,17.3 JP81.1
N$117  (via drill 0.3)
  Top 0.152: v37.26,25.38 37.26,27.81 39.47,30.02 39.93,30.02 40.16,29.79 41.45,29.79 IC5.2 | v33,25.15 18.44,25.15 18.21,24.92 JP82.1
  Bottom 0.152: v37.26,25.38 33.22,25.38 v33,25.15
N$118  (via drill 0.3)
  Top 0.152: v48.92,31.01 46.71,31.01 44.2,28.5 41.53,28.5 IC5.4 | v51.05,28.73 51.51,28.73 55.32,24.92 57.23,24.92 JP83.1
  Bottom 0.152: v48.92,31.01 48.92,30.86 v51.05,28.73
N$119
  Top 0.152: IC3.13 47.17,37.57 52.88,37.57 56.77,33.68 58.45,33.68 59.59,32.54 70.18,32.54 JP84.1
N$120  (via drill 0.3)
  Top 0.152: v67.97,33.22 67.82,33.07 66.07,33.07 60.35,38.79 53.11,38.79 51.66,40.23 46.79,40.23 46.41,39.85 46.41,38.63 46.79,38.25 47.09,38.25 IC3.14
  Bottom 0.152: v67.97,33.22 67.97,32.23 JP85.1
N$121  (via drill 0.3)
  Top 0.152: v58.83,34.21 58.83,35.43 57.84,36.42 55.02,36.42 52.58,38.86 47.17,38.86 IC3.15
  Bottom 0.152: v58.83,34.21 58.83,16.31 57.3,14.78 JP86.1
N$122
  Top 0.152: IC3.12 47.17,36.96 49.99,36.96 53.04,33.91 53.04,29.34 56.16,26.21 68.96,26.21 70.18,27.43 JP87.1
N$123
  Top 0.152: JP88.1 24.46,43.89 34.14,43.89 38.48,39.55 41.45,39.55 IC3.1
N$124  (via drill 0.3)
  Top 0.152: v39.62,37.03 40.54,37.03 40.62,36.96 41.45,36.96 IC3.5 | v43.66,27.13 43.66,26.98 41.38,24.69 36.2,24.69 27.89,16.38 19.81,16.38 JP89.1
  Bottom 0.152: v39.62,37.03 39.62,36.12 40.08,35.66 40.54,35.66 42.29,37.41 42.29,42.75 43.05,43.51 43.51,43.51 44.5,42.52 44.5,27.96 v43.66,27.13
N$125  (via drill 0.3)
  Top 0.152: v39.62,38.86 41.45,38.86 IC3.2 | v31.78,37.95 31.78,37.57 29.03,34.82 29.03,34.67 25.53,31.17 6.4,31.17 JP90.1
  Bottom 0.152: v39.62,38.86 32.69,38.86 v31.78,37.95
N$126  (via drill 0.3)
  Top 0.152: v31.09,43.2 34.37,43.2 39.93,37.64 41.45,37.64 IC3.4 | v28.73,45.57 20.04,45.57 8.99,34.52 7.24,34.52 5.26,32.54 JP91.1
  Bottom 0.152: v28.73,45.57 v31.09,43.2
N$127
  Top 0.152: R67.1 7.85,7.09 5.26,7.09 JP93.1
N$129
  Top 0.152: JP100.1 R47.2
N$130
  Top 0.152: R44.2 21.57,32.54 18.21,32.54 JP101.1
RESET  (via drill 0.3)
  Top 0.152: R45.1 6.1,76.73 6.1,77.34 7.39,78.64 SW2.B 7.47,78.72 14.17,78.72 SW2.B' 14.25,78.72 16,78.72 16.84,79.55 v29.19,79.55 | v38.48,75.89 38.48,77.04 IC10.7 38.41,77.11 38.41,79.32 37.03,80.7 v35.66,80.7 | v42.75,79.55 v45.34,79.55
  Bottom 0.152: v38.48,75.89 39.09,75.89 v42.75,79.55 | v29.19,79.55 34.22,79.55 35.36,80.7 v35.66,80.7 | v45.34,79.55 47.7,79.55 49.99,81.84 50.14,81.84 JP1.10
RIN  (via drill 0.3)
  Top 0.152: v72.24,63.78 68.28,67.74 67.44,67.74 IC12.19 | v65,5.87 58.6,5.87 55.78,3.05 C55.+
  Bottom 0.152: v72.24,63.78 72.24,42.9 72.39,42.75 72.39,12.65 70.56,10.82 69.72,10.82 65,6.1 v65,5.87
ROUT  (via drill 0.3)
  Top 0.152: v62.41,65.84 59.89,65.84 IC12.13 | v65.15,63.09 66.91,63.09 v73.61,56.39 | v13.87,3.35 12.42,3.35 12.12,3.05 C53.+
  Bottom 0.152: v65.15,63.09 v62.41,65.84 | v73.61,56.39 73.61,8.76 68.2,3.35 v13.87,3.35
RX  (via drill 0.3)
  Top 0.152: v40.46,61.87 43.74,61.87 44.27,62.41 44.27,65.61 42.75,67.13 40.23,67.13 39.02,65.91 39.02,65.3 IC10.43 | v34.67,57.61 32.62,57.61 v25.38,64.85
  Bottom 0.152: v40.46,61.87 40.01,61.87 39.7,62.18 39.24,62.18 v34.67,57.61 | v25.38,64.85 25.38,66.9 7.24,85.04 4.88,85.04 4.19,85.72 4.19,87.63 4.26,87.63 JP2.4
SW_GATE  (via drill 0.3)
  Top 0.152: v37.26,79.1 37.41,78.94 37.41,77.11 IC10.9 | v58.98,78.33 59.51,78.33 v61.72,76.12 | v71.4,31.55 70.94,31.55 70.56,31.17 61.04,31.17 57.3,27.43 JP94.1
  Bottom 0.152: v37.26,79.1 37.8,79.1 42.9,84.2 50.9,84.2 56.77,78.33 v58.98,78.33 | v61.72,76.12 61.72,75.67 61.49,75.44 61.49,67.67 65.84,63.32 65.84,46.1 70.64,41.3 70.79,41.3 71.4,40.69 v71.4,31.55
TX  (via drill 0.3)
  Top 0.152: v38.33,63.09 38.41,63.17 38.41,65.23 IC10.42
  Bottom 0.152: v38.33,63.09 37.87,63.09 37.26,62.48 30.02,62.48 27.81,64.69 27.81,66.45 10.44,83.82 8.92,83.82 6.55,86.18 5.45,86.18 JP2.5
VCC  (via drill 0.3)
  Top 0.305: 27.2,99.97 24,103.17 22.63,103.17 22.33,102.87 22.33,102.79 21.64,102.11 F1.2 21.57,102.03 21.57,97.69 13.79,89.92 12.35,89.92 C3.+ | 27.2,99.97 27.2,95.71 28.04,94.87 D1.- | v37.34,9.91 38.56,11.12 C44.1 | v38.48,8.76 40.08,8.76 40.31,8.99 IC14.8 | JP9.3 65.3,98.91 55.78,98.91 53.34,101.35 53.34,101.42 52.66,102.11 F2.2 52.5,102.03 50.52,100.05 27.28,100.05 27.2,99.97
  Bottom 0.305: v38.48,8.76 v37.34,9.91 37.41,9.98 37.41,12.8 55.86,31.24 55.86,40.92 63.17,48.23 63.17,59.44 60.81,61.8 60.81,91.67 JP9.3
VEE  (via drill 0.3)
  Top 0.305: 35.51,4.8 35.13,5.18 IC14.4 | 35.51,4.8 36.81,3.5 36.81,3.05 C45.2 | 68.89,84.81 68.89,85.8 R2.1 | 68.89,84.81 68.89,83.82 R1.1 | v51.13,97.46 50.45,98.15 47.93,98.15 D2.+ | v59.89,88.7 63.63,84.96 C1.- 63.7,84.81 68.89,84.81 | 35.51,4.8 36.88,6.17 v36.88,7.16
  Bottom 0.305: v51.13,97.46 v59.89,88.7 60.2,88.39 60.2,61.49 62.56,59.13 62.56,48.54 55.25,41.22 55.25,31.55 36.42,12.72 36.42,9.53 36.88,9.07 v36.88,7.16

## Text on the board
bPlace: JACK LIGHTS | ON | OFF | POWER | V1.0 | ATOM | ANTUMBRA | WWW.ANTUMBRA.EU
tNames: RESET | SYSBOOT
bNames: SERIAL | GND | <TX | JTAG | Original design by: Olivier Gillet / Redesign by: David Szebenyi / cc-by-sa Olivier Gillet, 2014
